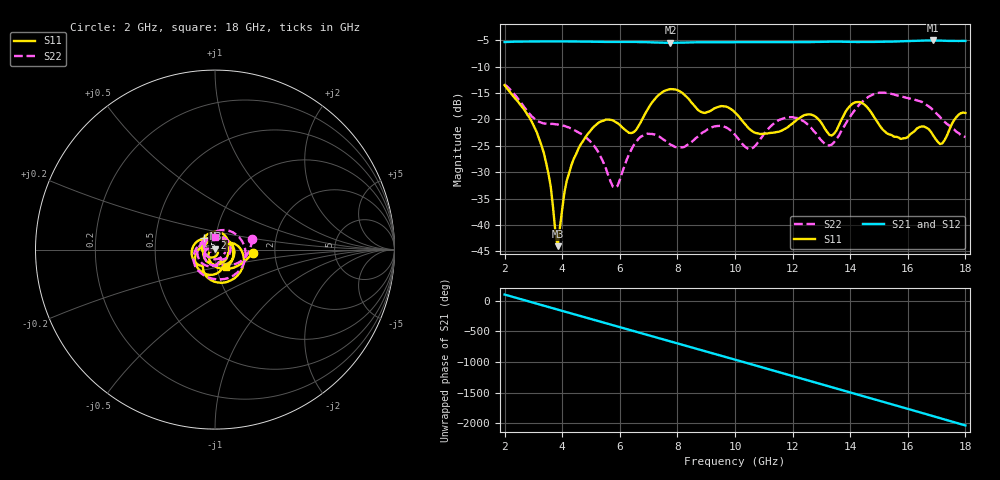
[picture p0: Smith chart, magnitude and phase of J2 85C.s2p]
!Agilent Technologies,E8363B,SG43030131,A.07.50.48
!Agilent E8363B: A.07.50.48
!Date: Wednesday, December 17, 2025 22:39:55
!Correction: S11(Full 2 Port(1,2))
!S21(Full 2 Port(1,2))
!S12(Full 2 Port(1,2))
!S22(Full 2 Port(1,2))
!S2P File: Measurements: S11, S21, S12, S22:
# Hz S  dB  R 50
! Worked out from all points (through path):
!   201 points, 2 GHz to 18 GHz, reference 50 ohm
!   highest |S21| = -5.06 dB at 16.88 GHz (marker M1); lowest = -5.5 dB at 7.76 GHz (marker M2)
!   group delay of S21, straight-line fit = 370 ps
!   lowest |S11| = -44.0 dB at 3.84 GHz (marker M3), VSWR 1.01, Z = 50.2 + j0.581 ohm
!   |S11| at or under -10 dB: start of sweep to end of sweep
!   |S22| runs from -32.9 to -13.4 dB; largest |S21 - S12| = 0.0024
!   S11 on the Smith chart (normalised r, x): 2 GHz: 1.53, -0.06; 5.2 GHz: 0.88, +0.12; 18 GHz: 1.11, -0.22
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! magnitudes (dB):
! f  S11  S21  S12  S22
! 2 GHz  -13.5  -5.4  -5.4  -13.4
! 3.28 GHz  -24.9  -5.2  -5.2  -20.6
! 3.6 GHz  -32.7  -5.2  -5.2  -20.9
! 3.84 GHz  -44.0  -5.2  -5.2  -21.0
! 4.16 GHz  -31.6  -5.2  -5.2  -21.4
! 4.72 GHz  -24.1  -5.3  -5.3  -23.0
! 5.2 GHz  -20.9  -5.3  -5.3  -25.7
! 5.84 GHz  -20.5  -5.3  -5.3  -32.9
! 6.48 GHz  -22.4  -5.3  -5.3  -24.9
! 7.36 GHz  -15.3  -5.5  -5.5  -23.2
! 7.76 GHz  -14.3  -5.5  -5.5  -24.8
! 10 GHz  -18.7  -5.4  -5.4  -22.9
! 10.48 GHz  -21.7  -5.4  -5.4  -25.6
! 10.88 GHz  -22.8  -5.4  -5.4  -23.7
! 11.84 GHz  -21.5  -5.4  -5.4  -19.6
! 12.72 GHz  -19.2  -5.4  -5.4  -22.1
! 13.36 GHz  -23.1  -5.3  -5.3  -24.8
! 14.32 GHz  -16.7  -5.4  -5.4  -17.2
! 15.36 GHz  -22.8  -5.3  -5.3  -15.1
! 16.88 GHz  -23.0  -5.1  -5.1  -18.3
! 17.2 GHz  -24.5  -5.1  -5.1  -20.1
! 18 GHz  -18.8  -5.1  -5.1  -23.4
